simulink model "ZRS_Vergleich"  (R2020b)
settings: Solver=ode3  StartTime=0.0  StopTime=2  FixedStep=1e-4  RelTol=1e-8  EnableMultiTasking=on
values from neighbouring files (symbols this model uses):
  A = [0 1; -w0^2 -2*delta]    [parameter.m]    (also in finite_differences.m = diag(coeff1*ones(1,N(i))) +          diag(coeff2*ones(1,N(i); viertelfahrzeugmodell.m = [0          0      1     0)
  B = [0; 1/m]    [parameter.m]    (also in viertelfahrzeugmodell.m = [0)
  Bz = B    [parameter.m]
  C = [1 0]    [parameter.m]    (also in viertelfahrzeugmodell.m = [1  0  0  0])
undefined symbols (not defined in the file or in its folder): ZR, ZRPI, ZRS

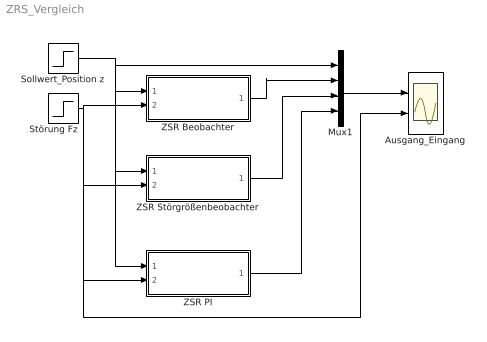
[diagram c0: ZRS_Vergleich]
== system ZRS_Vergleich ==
  Ausgang_Eingang : Scope  NumInputPorts=2
  Mux1 : Mux
  Sollwert_Position z : Step  Time=0.1  SampleTime=0
  Störung Fz : Step  After=5  SampleTime=0
  ZSR Beobachter : Subsystem
  ZSR PI : Subsystem
  ZSR Störgrößenbeobachter : Subsystem
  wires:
  Störung Fz/1 -> ZSR Beobachter/2(z), Ausgang_Eingang/2, ZSR PI/2(z), ZSR Störgrößenbeobachter/2(z)
  Sollwert_Position z/1 -> Mux1/1, ZSR PI/1(w), ZSR Störgrößenbeobachter/1(w), ZSR Beobachter/1(w)
  Mux1/1 -> Ausgang_Eingang/1
  ZSR Beobachter/1(v) -> Mux1/2
  ZSR Störgrößenbeobachter/1(v) -> Mux1/3
  ZSR PI/1(v) -> Mux1/4

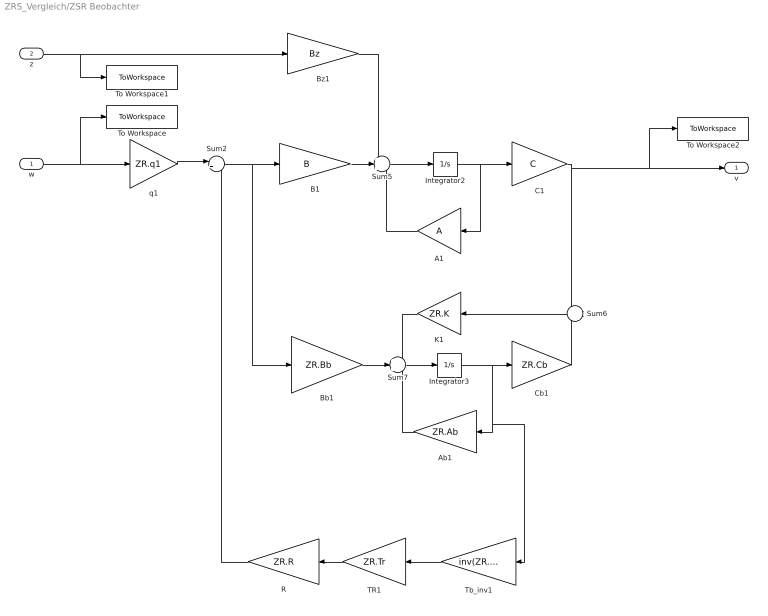
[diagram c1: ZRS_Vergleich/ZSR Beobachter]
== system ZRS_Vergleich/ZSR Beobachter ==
  w : Inport
  z : Inport  Port=2
  A1 : Gain  Gain=A  Multiplication=Matrix(K*u) (u vector)
  Ab1 : Gain  Gain=ZR.Ab  Multiplication=Matrix(K*u) (u vector)
  B1 : Gain  Gain=B  Multiplication=Matrix(K*u) (u vector)
  Bb1 : Gain  Gain=ZR.Bb  Multiplication=Matrix(K*u) (u vector)
  Bz1 : Gain  Gain=Bz  Multiplication=Matrix(K*u) (u vector)
  C1 : Gain  Gain=C  Multiplication=Matrix(K*u) (u vector)
  Cb1 : Gain  Gain=ZR.Cb  Multiplication=Matrix(K*u) (u vector)
  Integrator2 : Integrator
  Integrator3 : Integrator
  K1 : Gain  Gain=ZR.K  Multiplication=Matrix(K*u) (u vector)
  R : Gain  Gain=ZR.R  Multiplication=Matrix(K*u) (u vector)
  Sum2 : Sum  Inputs=|+-
  Sum5 : Sum  Inputs=+++
  Sum6 : Sum  Inputs=+|-
  Sum7 : Sum  Inputs=+++
  TR1 : Gain  Gain=ZR.Tr  Multiplication=Matrix(K*u) (u vector)
  Tb_inv1 : Gain  Gain=inv(ZR.Tb)  Multiplication=Matrix(K*u) (u vector)
  To Workspace : ToWorkspace  VariableName=w  SaveFormat=Timeseries  SampleTime=-1
  To Workspace1 : ToWorkspace  VariableName=z  SaveFormat=Timeseries  SampleTime=-1
  To Workspace2 : ToWorkspace  VariableName=out1  SaveFormat=Timeseries  SampleTime=-1
  q1 : Gain  Gain=ZR.q1  Multiplication=Matrix(K*u)
  v : Outport
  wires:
  w/1 -> To Workspace/1, q1/1
  q1/1 -> Sum2/1
  Sum2/1 -> Bb1/1, B1/1
  Sum5/1 -> Integrator2/1
  Integrator2/1 -> C1/1, A1/1
  C1/1 -> Sum6/1, To Workspace2/1, v/1
  Sum6/1 -> K1/1
  Sum7/1 -> Integrator3/1
  Integrator3/1 -> Cb1/1, Ab1/1, Tb_inv1/1
  K1/1 -> Sum7/1
  Bb1/1 -> Sum7/2
  Ab1/1 -> Sum7/3
  Cb1/1 -> Sum6/2
  R/1 -> Sum2/2
  Bz1/1 -> Sum5/1
  B1/1 -> Sum5/2
  A1/1 -> Sum5/3
  TR1/1 -> R/1
  Tb_inv1/1 -> TR1/1
  z/1 -> To Workspace1/1, Bz1/1

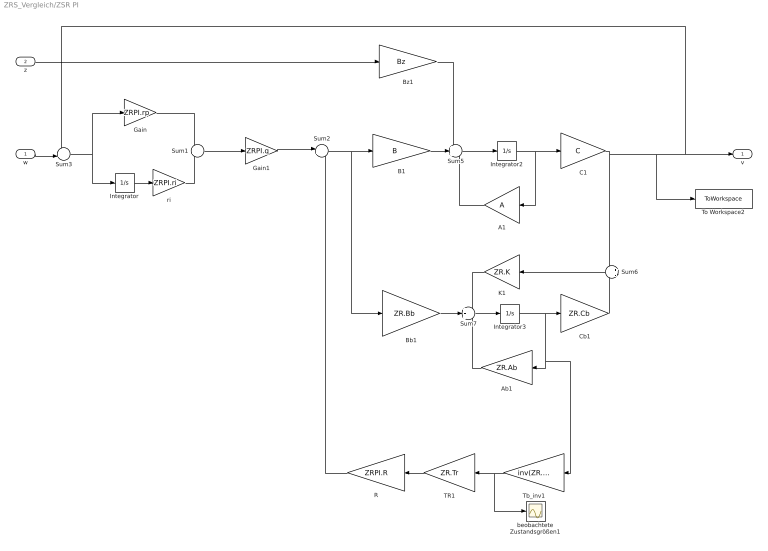
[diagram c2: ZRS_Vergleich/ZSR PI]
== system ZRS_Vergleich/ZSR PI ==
  w : Inport
  z : Inport  Port=2
  A1 : Gain  Gain=A  Multiplication=Matrix(K*u) (u vector)
  Ab1 : Gain  Gain=ZR.Ab  Multiplication=Matrix(K*u) (u vector)
  B1 : Gain  Gain=B  Multiplication=Matrix(K*u) (u vector)
  Bb1 : Gain  Gain=ZR.Bb  Multiplication=Matrix(K*u) (u vector)
  Bz1 : Gain  Gain=Bz  Multiplication=Matrix(K*u) (u vector)
  C1 : Gain  Gain=C  Multiplication=Matrix(K*u) (u vector)
  Cb1 : Gain  Gain=ZR.Cb  Multiplication=Matrix(K*u) (u vector)
  Gain : Gain  Gain=ZRPI.rp  Multiplication=Matrix(K*u)
  Gain1 : Gain  Gain=ZRPI.q  Multiplication=Matrix(K*u)
  Integrator : Integrator
  Integrator2 : Integrator
  Integrator3 : Integrator
  K1 : Gain  Gain=ZR.K  Multiplication=Matrix(K*u) (u vector)
  R : Gain  Gain=ZRPI.R  Multiplication=Matrix(K*u) (u vector)
  Sum1 : Sum
  Sum2 : Sum  Inputs=|+-
  Sum3 : Sum  Inputs=-+|
  Sum5 : Sum  Inputs=+++
  Sum6 : Sum  Inputs=+|-
  Sum7 : Sum  Inputs=+++
  TR1 : Gain  Gain=ZR.Tr  Multiplication=Matrix(K*u) (u vector)
  Tb_inv1 : Gain  Gain=inv(ZR.Tb)  Multiplication=Matrix(K*u) (u vector)
  To Workspace2 : ToWorkspace  VariableName=out3  SaveFormat=Timeseries  SampleTime=-1
  beobachtete Zustandsgrößen1 : Scope
  ri : Gain  Gain=ZRPI.ri  Multiplication=Matrix(K*u)
  v : Outport
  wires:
  z/1 -> Bz1/1
  Tb_inv1/1 -> beobachtete Zustandsgrößen1/1, TR1/1
  TR1/1 -> R/1
  A1/1 -> Sum5/3
  B1/1 -> Sum5/2
  Bz1/1 -> Sum5/1
  R/1 -> Sum2/2
  Cb1/1 -> Sum6/2
  Ab1/1 -> Sum7/3
  Bb1/1 -> Sum7/2
  K1/1 -> Sum7/1
  Integrator3/1 -> Tb_inv1/1, Ab1/1, Cb1/1
  Sum7/1 -> Integrator3/1
  Sum6/1 -> K1/1
  C1/1 -> Sum6/1, To Workspace2/1, v/1, Sum3/1
  Integrator2/1 -> A1/1, C1/1
  Sum5/1 -> Integrator2/1
  Sum2/1 -> B1/1, Bb1/1
  Sum3/1 -> Gain/1, Integrator/1
  Gain/1 -> Sum1/1
  ri/1 -> Sum1/2
  Integrator/1 -> ri/1
  w/1 -> Sum3/2
  Sum1/1 -> Gain1/1
  Gain1/1 -> Sum2/1

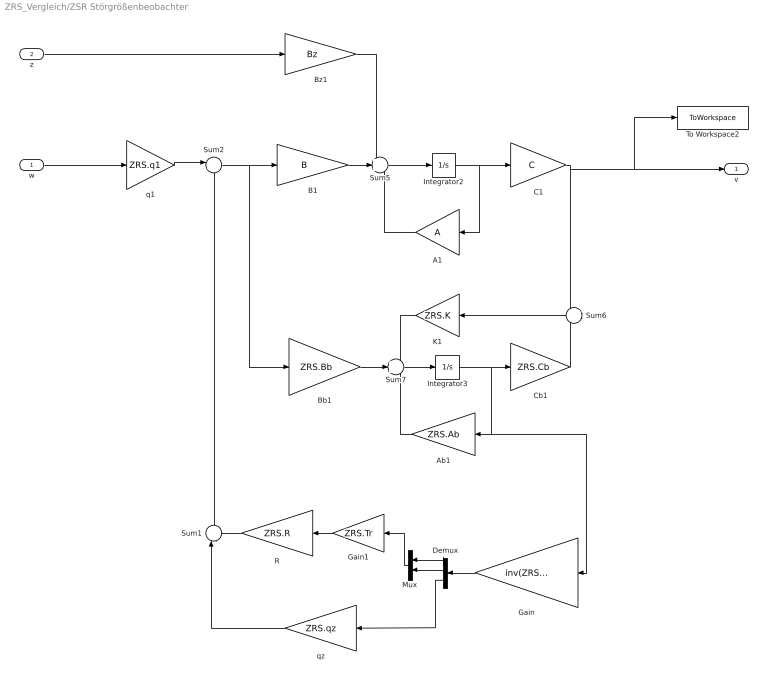
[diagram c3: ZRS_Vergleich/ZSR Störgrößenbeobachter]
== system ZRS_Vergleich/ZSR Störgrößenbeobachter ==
  w : Inport
  z : Inport  Port=2
  A1 : Gain  Gain=A  Multiplication=Matrix(K*u) (u vector)
  Ab1 : Gain  Gain=ZRS.Ab  Multiplication=Matrix(K*u) (u vector)
  B1 : Gain  Gain=B  Multiplication=Matrix(K*u) (u vector)
  Bb1 : Gain  Gain=ZRS.Bb  Multiplication=Matrix(K*u) (u vector)
  Bz1 : Gain  Gain=Bz  Multiplication=Matrix(K*u) (u vector)
  C1 : Gain  Gain=C  Multiplication=Matrix(K*u) (u vector)
  Cb1 : Gain  Gain=ZRS.Cb  Multiplication=Matrix(K*u) (u vector)
  Demux : Demux  Outputs=3
  Gain : Gain  Gain=inv(ZRS.Tb)  Multiplication=Matrix(K*u)
  Gain1 : Gain  Gain=ZRS.Tr  Multiplication=Matrix(K*u)
  Integrator2 : Integrator
  Integrator3 : Integrator
  K1 : Gain  Gain=ZRS.K  Multiplication=Matrix(K*u) (u vector)
  Mux : Mux  Inputs=2
  R : Gain  Gain=ZRS.R  Multiplication=Matrix(K*u) (u vector)
  Sum1 : Sum  Inputs=|-+
  Sum2 : Sum  Inputs=|+-
  Sum5 : Sum  Inputs=+++
  Sum6 : Sum  Inputs=+|-
  Sum7 : Sum  Inputs=+++
  To Workspace2 : ToWorkspace  VariableName=out2  SaveFormat=Timeseries  SampleTime=-1
  q1 : Gain  Gain=ZRS.q1  Multiplication=Matrix(K*u)
  qz : Gain  Gain=ZRS.qz  Multiplication=Matrix(K*u) (u vector)
  v : Outport
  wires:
  z/1 -> Bz1/1
  A1/1 -> Sum5/3
  B1/1 -> Sum5/2
  Bz1/1 -> Sum5/1
  Cb1/1 -> Sum6/2
  Ab1/1 -> Sum7/3
  Bb1/1 -> Sum7/2
  K1/1 -> Sum7/1
  Integrator3/1 -> Cb1/1, Ab1/1, Gain/1
  Sum7/1 -> Integrator3/1
  Sum6/1 -> K1/1
  C1/1 -> To Workspace2/1, v/1, Sum6/1
  Integrator2/1 -> A1/1, C1/1
  Sum5/1 -> Integrator2/1
  Sum2/1 -> B1/1, Bb1/1
  q1/1 -> Sum2/1
  w/1 -> q1/1
  R/1 -> Sum1/2
  qz/1 -> Sum1/1
  Sum1/1 -> Sum2/2
  Gain/1 -> Demux/1
  Demux/1 -> Mux/1
  Demux/2 -> Mux/2
  Demux/3 -> qz/1
  Gain1/1 -> R/1
  Mux/1 -> Gain1/1
